PROGRAM p01_spreminjanjeVI
VAR
	S0 AT %I*: BOOL;
	S1 AT %I*: BOOL;
	L0 AT %Q*: BOOL;
	L1 AT %Q*: BOOL;
END_VAR

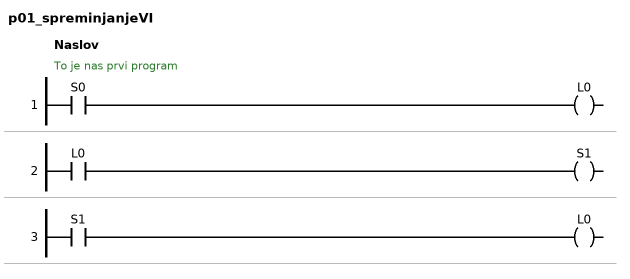
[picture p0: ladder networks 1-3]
// NETWORK 1: Naslov
// To je nas prvi program
L0 := S0;

// NETWORK 2
S1 := L0;

// NETWORK 3
L0 := S1;

END_PROGRAM
